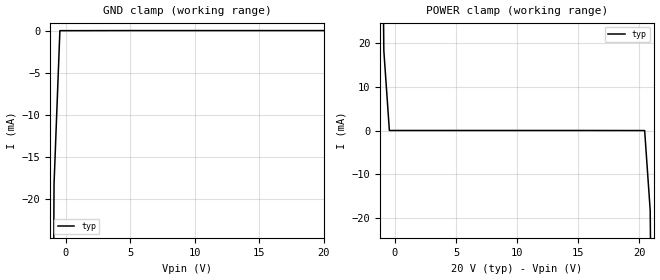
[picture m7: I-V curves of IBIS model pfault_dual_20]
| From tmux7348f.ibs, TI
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| pfault_dual_20
[Model]   pfault_dual_20
Model_type   Input
Vinl = 0.8
Vinh = 1.3
|   typ   min   max
C_comp   1.008417e-11   NA   NA
[Voltage Range]   20   NA   NA
[Temperature Range]   27   NA   NA
[Power Clamp Reference]   20   NA   NA
[GND Clamp Reference]   0   NA   NA
[GND Clamp]
|   Voltage   I(typ)   I(min)   I(max)
-25V      -35.96A    NA         NA
-1.364V   -155.4mA   NA         NA
-909.1mV  -18.23mA   NA         NA
-454.5mV  -235.8nA   NA         NA
20V       9.994uA    NA         NA
[POWER Clamp]
|   Voltage   I(typ)   I(min)   I(max)
-5V       1.413A     NA         NA
-1.364V   155.3mA    NA         NA
-909.1mV  18.23mA    NA         NA
-454.5mV  10.01uA    NA         NA
20.45V    -235.8nA   NA         NA
20.91V    -18.23mA   NA         NA
21.36V    -155.4mA   NA         NA
40V       -7.855A    NA         NA
